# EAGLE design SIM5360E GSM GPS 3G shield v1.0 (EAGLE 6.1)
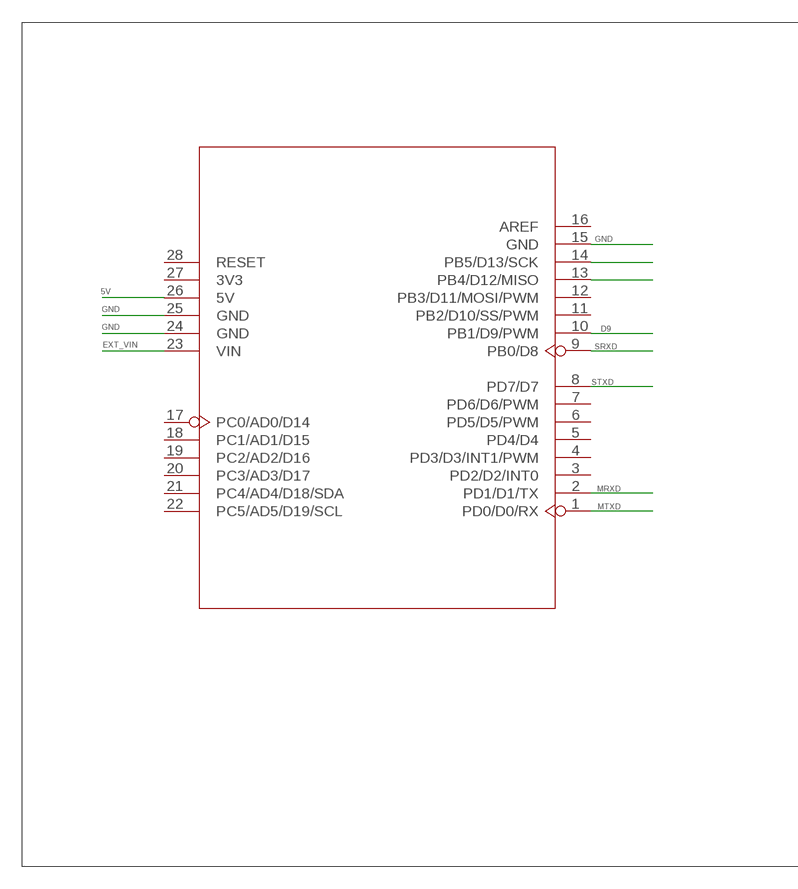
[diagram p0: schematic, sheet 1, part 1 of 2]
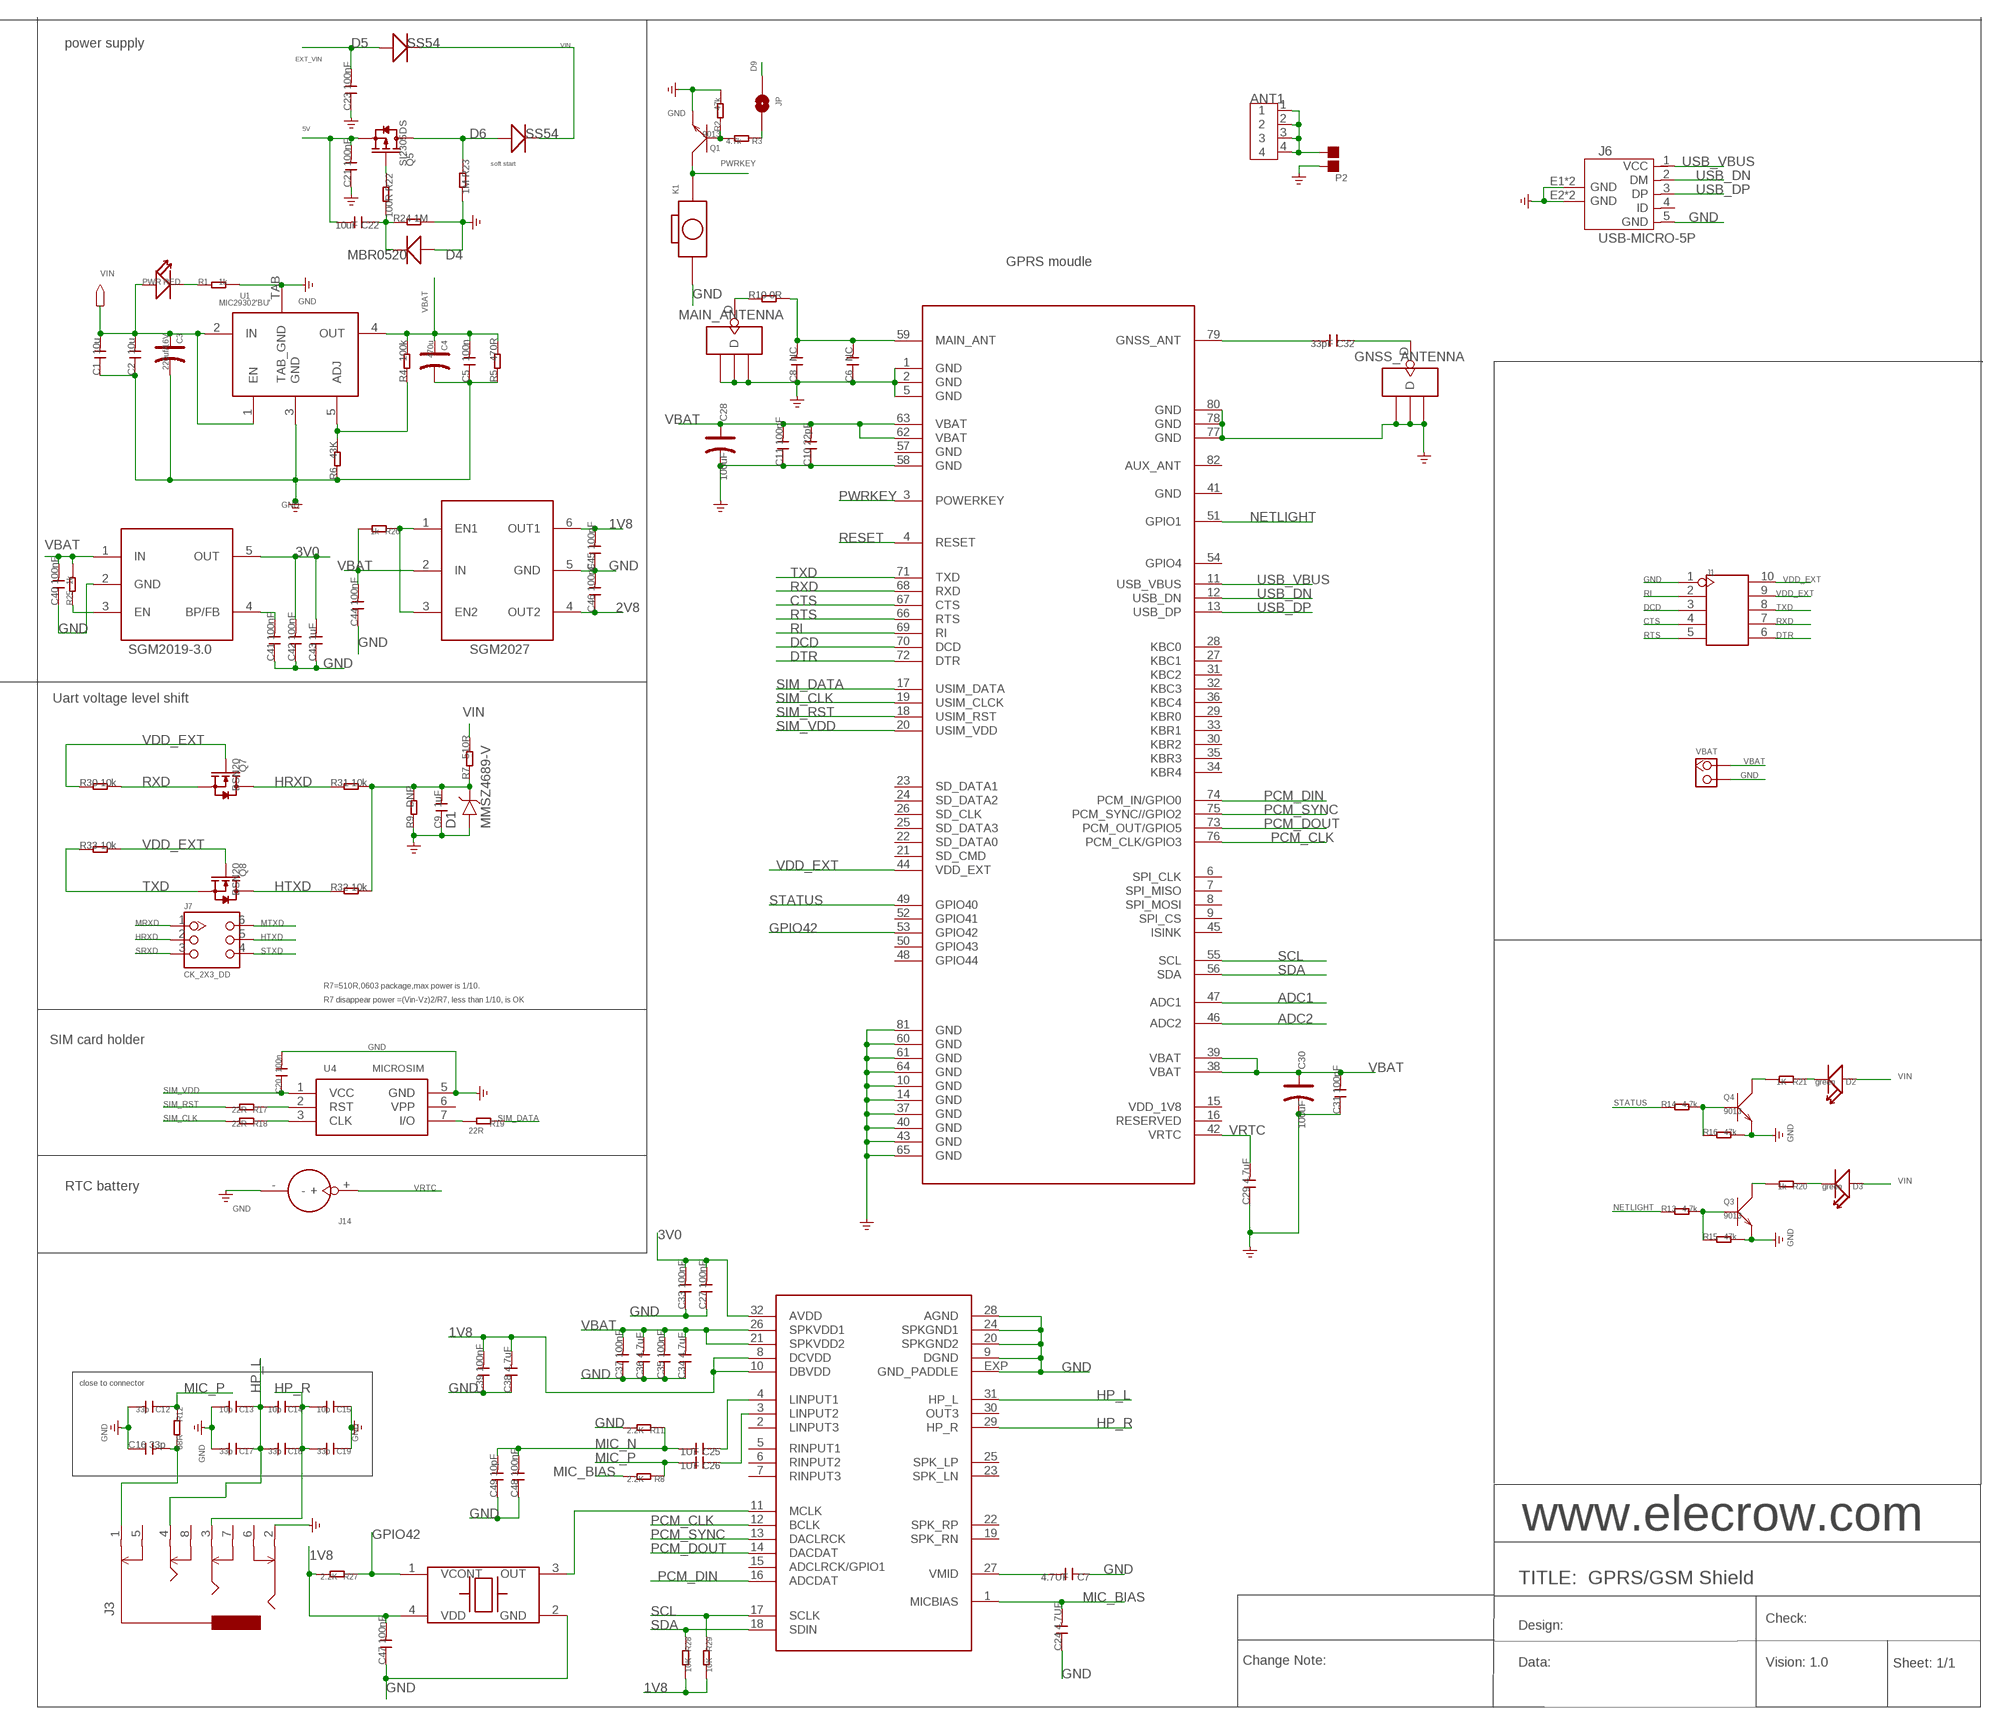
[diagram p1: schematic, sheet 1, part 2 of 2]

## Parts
ANT1  ANTENNA-SMA-IPX  [SMA-TO-IPX]
C1  10u  C-0603  [C0603]
C2  10u  C-0603  [C0603]
C3  220uf/16V  006-CAP_AVX_D  [AVX_D]
C4  470u  006-CAP_AVX_D  [AVX_D]
C5  100n  C-0603  [C0603]
C6  NC  C-0603  [C0603]
C7  4.7UF  C-0603  [C0603]
C8  NC  C-0603  [C0603]
C9  1uF  C-0603  [C0603]
C10  22pF  C-0603  [C0603]
C11  100nF  C-0603  [C0603]
C12  33p  C-0603  [C0603]
C13  10p  C-0402  [C0402]
C14  10p  C-0402  [C0402]
C15  10p  C-0402  [C0402]
C16  33p  C-0603  [C0603]
C17  33p  C-0402  [C0402]
C18  33p  C-0402  [C0402]
C19  33p  C-0402  [C0402]
C20  100n  C-0603  [C0603]
C21  100nF  C-0603  [C0603]
C22  10uF  C-0805  [C0805]
C23  100nF  C-0603  [C0603]
C24  4.7UF  C-0603  [C0603]
C25  1UF  C-0603  [C0603]
C26  1UF  C-0603  [C0603]
C27  100nF  C-0603  [C0603]
C28  100uF  CAP-AVX-B  [AVX-B]
C29  4.7uF  C-0805  [C0805]
C30  100uF  CAP-AVX-B  [AVX-B]
C31  100nF  C-0603  [C0603]
C32  33pF  C-0603  [C0603]
C33  100nF  C-0603  [C0603]
C34  4.7uF  C-0603  [C0603]
C35  100nF  C-0603  [C0603]
C36  4.7uF  C-0603  [C0603]
C37  100nF  C-0603  [C0603]
C38  4.7uF  C-0603  [C0603]
C39  100nF  C-0603  [C0603]
C40  100nF  C-0603  [C0603]
C41  100nF  C-0603  [C0603]
C42  100nF  C-0603  [C0603]
C43  1uF  C-0603  [C0603]
C44  100nF  C-0603  [C0603]
C45  100nF  C-0603  [C0603]
C46  100nF  C-0603  [C0603]
C47  100nF  C-0603  [C0603]
C48  100nF  C-0603  [C0603]
C49  10pF  C-0603  [C0603]
D1  MMSZ4689-V  D-VOL'MMSZ4681'  [SOD123-2.7X1.6]
D2  green  LED'0603'  [LED-0603]
D3  green  LED'0603'  [LED-0603]
D4  MBR0520  D'MBR0520LT1'  [SOD123-2.7X1.6]
D5  SS54  D'MBRS240LT3'  [SMB]
D6  SS54  D'MBRS240LT3'  [SMB]
GNSS_ANTENNA  ANTENNA-U-FL  [4P-U-FL]
J1  HEADER-2X5P-2.54  [2X5P-2.54]
J3  AUDIO-8P'PJ-3536-L6S'  [8P-3.5-SMD]
J6  USB-MICRO-5P  [MICRO-USB-5P]
J7  CK_2X3_DD  [CK_2X3]
J14  HOLDER-BATTERY-2P-CR1220  [CR1220]
JP  0R/0805  PAD-SOLDERJUMPERNC  [2P-SMD-3.3X2]
K1  BOTTON_1_DP  [BTN_5.0_RST]
MAIN_ANTENNA  ANTENNA-U-FL  [4P-U-FL]
P2  PAD-JUMPER-2P  [2P-SMD-1.78X1.27]
PWR  RED  007-LED0603  [D0603]
Q1  9013  TRANSISTOR-NPN-SOT23  [SOT23]
Q3  9013  TRANSISTOR-NPN-SOT23  [SOT23]
Q4  9013  TRANSISTOR-NPN-SOT23  [SOT23]
Q5  SI2305DS  MOSFET-P'SI2323CDS/SI2305DS<BR>'  [SOT23]
Q7  BSN20  MOSFET-N'SOT23'  [SOT23]
Q8  BSN20  MOSFET-N'SOT23'  [SOT23]
R1  1k  R-0603  [R0603]
R2  47k  R-0603  [R0603]
R3  4.7k  R-0603  [R0603]
R4  100k  R-0603  [R0603]
R5  470R  R-0603  [R0603]
R6  43K  R-0603  [R0603]
R7  510R  R-0603  [R0603]
R8  2.2K  R-0603  [R0603]
R9  DNP  R-0603  [R0603]
R10  0R  R-0603  [R0603]
R11  2.2K  R-0603  [R0603]
R12  68R  R-0603  [R0603]
R13  4.7k  R-0603  [R0603]
R14  4.7k  R-0603  [R0603]
R15  47k  R-0603  [R0603]
R16  47k  R-0603  [R0603]
R17  22R  R-0603  [R0603]
R18  22R  R-0603  [R0603]
R19  22R  R-0603  [R0603]
R20  1k  R-0603  [R0603]
R21  1K  R-0603  [R0603]
R22  100R  R-0603  [R0603]
R23  1M  R-0603  [R0603]
R24  1M  R-0603  [R0603]
R25  1k  R-0603  [R0603]
R26  1k  R-0603  [R0603]
R27  2.2K  R-0603  [R0603]
R28  10K  R-0603  [R0603]
R29  10K  R-0603  [R0603]
R30  10k  R-0603  [R0603]
R31  10k  R-0603  [R0603]
R32  10k  R-0603  [R0603]
R33  10k  R-0603  [R0603]
U1  MIC29302'BU'  [TO-263]
U3  UNO-SHILED  [SHILED]
U4  MICROSIM  [MICROSIM]
U5  VM8960GEFL  [QFN32-4.9X4.9]
U12  SGM2027  [TSOT6]
U21  SGM2019  [SOT23-5]
U26  8W26000011  [8W2600001]
U$8  SIM5360E  [SIM5360]
VBAT  DNP  HEADER_1X2_2.54  [CK_1*2]

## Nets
1V8: C38.2 C39.2 C45.2 C47.2 R27.2 R28.2 R29.2 U5.8(DCVDD) U5.10(DBVDD) U12.6(OUT1) U26.4(VDD)
2V8: C46.1 U12.4(OUT2)
3V0: C27.2 C33.2 C42.2 C43.2 U5.32(AVDD) U21.5(OUT)
5V: C21.2 C22.2 Q5.2(S) U3.26(5V)
ADC1: U$8.47(ADC1)
ADC2: U$8.46(ADC2)
CTS: J1.4 U$8.67(CTS)
D9: JP.1 U3.10(PB1/D9/PWM)
DCD: J1.3 U$8.70(DCD)
DTR: J1.6 U$8.72(DTR)
EXT_VIN: C23.2 D5.+ U3.23(VIN)
GND: C1.1 C2.1 C3.- C4.- C5.1 C6.1 C7.1 C8.1 C9.1 C10.1 C11.1 C12.2 C13.2 C15.1 C16.1 C17.2 C19.1 C20.2 C21.1 C23.1 C24.1 C27.1 C28.- C29.1 C30.- C31.1 C33.1 C34.1 C35.1 C36.1 C37.1 C38.1 C39.1 C40.1 C41.1 C42.1 C43.1 C44.1 C46.2 C47.1 C48.1 C49.1 D1.1 D4.1(+) GNSS_ANTENNA.GND1 GNSS_ANTENNA.GND2 GNSS_ANTENNA.GND3 J1.1 J3.2 J6.5(GND) J6.E1(GND) J6.E2(GND) J6.P1(GND) J6.P2(GND) J14.- K1.P$1 MAIN_ANTENNA.GND1 MAIN_ANTENNA.GND2 MAIN_ANTENNA.GND3 P2.2 Q1.2(E) Q3.2(E) Q4.2(E) R1.2 R2.2 R5.1 R6.1 R9.1 R11.2 R15.2 R16.2 R23.2 R24.2 U1.3(GND) U1.TAB(TAB_GND) U3.15(GND) U3.24(GND) U3.25(GND) U4.5(GND) U5.9(DGND) U5.20(SPKGND2) U5.24(SPKGND1) U5.28(AGND) U5.EXP(GND_PADDLE) U12.5(GND) U21.2(GND) U26.2(GND) U$8.1(GND) U$8.2(GND) U$8.5(GND) U$8.10(GND) U$8.14(GND) U$8.37(GND) U$8.40(GND) U$8.43(GND) U$8.58(GND) U$8.60(GND) U$8.61(GND) U$8.64(GND) U$8.65(GND) U$8.77(GND) U$8.78(GND) U$8.80(GND) U$8.81(GND) VBAT.2
GPIO42: R27.1 U26.1(VCONT) U$8.53(GPIO42)
HP_L: C13.1 C14.2 C17.1 C18.2 J3.4 U5.31(HP_L)
HP_R: C14.1 C15.2 C18.1 C19.2 J3.3 U5.29(HP_R)
HRXD: J7.2 Q7.3(D) R31.1
HTXD: J7.5 Q8.3(D) R32.1
MIC_BIAS: C24.2 R8.2 U5.1(MICBIAS)
MIC_N: C25.2 C48.2 C49.2 R11.1
MIC_P: C12.1 C26.2 R8.1 R12.1
MRXD: J7.1 U3.2(PD1/D1/TX)
MTXD: J7.6 U3.1(PD0/D0/RX)
N$1: R19.2 U4.7(I/O)
N$2: R4.1 R6.2 U1.5(ADJ)
N$3: Q3.3(C) R20.2
N$4: C7.2 U5.27(VMID)
N$5: R18.1 U4.3(CLK)
N$6: R17.1 U4.2(RST)
N$7: D3.- R20.1
N$8: Q3.1(B) R13.2 R15.1
N$9: C9.2 D1.2 R7.1 R9.2 R31.2 R32.2
N$11: Q5.1(G) R22.1
N$12: ANT1.1 ANT1.2 ANT1.3 ANT1.4 P2.1
N$13: U5.11(MCLK) U26.3(OUT)
N$14: JP.2 R3.1
N$15: C6.2 C8.2 R10.2 U$8.59(MAIN_ANT)
N$16: Q4.3(C) R21.2
N$17: D2.- R21.1
N$18: Q4.1(B) R14.2 R16.1
N$19: MAIN_ANTENNA.D R10.1
N$20: D6.+ Q5.3(D) R23.1
N$21: C25.1 U5.4(LINPUT1)
N$22: C26.1 U5.3(LINPUT2)
N$23: U3.14(PB5/D13/SCK)
N$25: C41.2 U21.4(BP/FB)
N$26: R25.1 U21.3(EN)
N$27: U3.13(PB4/D12/MISO)
N$28: R26.1 U12.1(EN1) U12.3(EN2)
N$30: C16.2 J3.1 R12.2
N$36: Q1.1(B) R2.1 R3.2
N$39: C22.1 D4.2(-) R22.2 R24.1
N$53: PWR.- R1.1
N$54: C32.2 U$8.79(GNSS_ANT)
N$55: C32.1 GNSS_ANTENNA.D
NETLIGHT: R13.1 U$8.51(GPIO1)
PCM_CLK: U5.12(BCLK) U$8.76(PCM_CLK/GPIO3)
PCM_DIN: U5.16(ADCDAT) U$8.74(PCM_IN/GPIO0)
PCM_DOUT: U5.14(DACDAT) U$8.73(PCM_OUT/GPIO5)
PCM_SYNC: U5.13(DACLRCK) U$8.75(PCM_SYNC//GPIO2)
PWRKEY: K1.P$2 Q1.3(C) U$8.3(POWERKEY)
RESET: U$8.4(RESET)
RI: J1.2 U$8.69(RI)
RTS: J1.5 U$8.66(RTS)
RXD: J1.7 Q7.2(S) R30.2 U$8.68(RXD)
SCL: R29.1 U5.17(SCLK) U$8.55(SCL)
SDA: R28.1 U5.18(SDIN) U$8.56(SDA)
SIM_CLK: R18.2 U$8.19(USIM_CLCK)
SIM_DATA: R19.1 U$8.17(USIM_DATA)
SIM_RST: R17.2 U$8.18(USIM_RST)
SIM_VDD: C20.1 U4.1(VCC) U$8.20(USIM_VDD)
SRXD: J7.3 U3.9(PB0/D8)
STATUS: R14.1 U$8.49(GPIO40)
STXD: J7.4 U3.8(PD7/D7)
TXD: J1.8 Q8.2(S) R33.1 U$8.71(TXD)
USB_DN: J6.2(DM) U$8.12(USB_DN)
USB_DP: J6.3(DP) U$8.13(USB_DP)
USB_VBUS: J6.1(VCC) U$8.11(USB_VBUS)
VBAT: C4.+ C5.2 C10.2 C11.2 C28.+ C30.+ C31.2 C34.2 C35.2 C36.2 C37.2 C40.2 C44.2 R4.2 R5.2 R25.2 R26.2 U1.4(OUT) U5.21(SPKVDD2) U5.26(SPKVDD1) U12.2(IN) U21.1(IN) U$8.38(VBAT) U$8.39(VBAT) U$8.62(VBAT) U$8.63(VBAT) VBAT.1
VDD_EXT: J1.9 J1.10 Q7.1(G) Q8.1(G) R30.1 R33.2 U$8.44(VDD_EXT)
VIN: C1.2 C2.2 C3.+ D2.+ D3.+ D5.- D6.- PWR.+ R7.2 U1.1(EN) U1.2(IN)
VRTC: C29.2 J14.+ U$8.42(VRTC)
Unconnected: C45.1 J3.5 J3.6 J3.7 J3.8 J6.4(ID) U3.3(PD2/D2/INT0) U3.4(PD3/D3/INT1/PWM) U3.5(PD4/D4) U3.6(PD5/D5/PWM) U3.7(PD6/D6/PWM) U3.11(PB2/D10/SS/PWM) U3.12(PB3/D11/MOSI/PWM) U3.16(AREF) U3.17(PC0/AD0/D14) U3.18(PC1/AD1/D15) U3.19(PC2/AD2/D16) U3.20(PC3/AD3/D17) U3.21(PC4/AD4/D18/SDA) U3.22(PC5/AD5/D19/SCL) U3.27(3V3) U3.28(RESET) U4.6(VPP) U5.2(LINPUT3) U5.5(RINPUT1) U5.6(RINPUT2) U5.7(RINPUT3) U5.15(ADCLRCK/GPIO1) U5.19(SPK_RN) U5.22(SPK_RP) U5.23(SPK_LN) U5.25(SPK_LP) U5.30(OUT3) U$8.6(SPI_CLK) U$8.7(SPI_MISO) U$8.8(SPI_MOSI) U$8.9(SPI_CS) U$8.15(VDD_1V8) U$8.16(RESERVED) U$8.21(SD_CMD) U$8.22(SD_DATA0) U$8.23(SD_DATA1) U$8.24(SD_DATA2) U$8.25(SD_DATA3) U$8.26(SD_CLK) U$8.27(KBC1) U$8.28(KBC0) U$8.29(KBR0) U$8.30(KBR2) U$8.31(KBC2) U$8.32(KBC3) U$8.33(KBR1) U$8.34(KBR4) U$8.35(KBR3) U$8.36(KBC4) U$8.41(GND) U$8.45(ISINK) U$8.48(GPIO44) U$8.50(GPIO43) U$8.52(GPIO41) U$8.54(GPIO4) U$8.57(GND) U$8.82(AUX_ANT)

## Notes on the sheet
- power supply
- soft start
- GPRS moudle
- SGM2019-3.0 | SGM2027
- Uart voltage level shift
- R7=510R,0603 package,max power is 1/10.
- R7 disappear power =(Vin-Vz)2/R7, less than 1/10, is OK
- SIM card holder
- RTC battery
- close to connector
- www.elecrow.com
- TITLE:  GPRS/GSM Shield
- Check:
- Design:
- Change Note: | Data: | Vision: 1.0 | Sheet: 1/1

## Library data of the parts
ANT1 = Connector:ANTENNA-SMA-IPX
C1 C2 C5-C27 C29 C31-C49 = Discrete:C*: Ceramic Capacitors
C3 C4 = Discrete:006-CAP*: Electrolytic Capacitors,Tantalum Capacitors and Super Capacitors
C28 C30 = Discrete:CAP*: Electrolytic Capacitors,Tantalum Capacitors and Super Capacitors
D1 = template:D-VOL
D2 D3 = Discrete:LED*
D4-D6 = Discrete:D*
GNSS_ANTENNA MAIN_ANTENNA = Connector:ANTENNA-U-FL
J1 = Connector:HEADER-2X5P
J3 = template:AUDIO-8P
J6 = Connector:USB-MICRO-5P
J7 = CONNECTER:CK_2X3
J14 = Connector:HOLDER-BATTERY-2P
JP = Discrete:PAD-SOLDERJUMPER: Solder Jumper
K1 = CPT_SMD:BOTTON_1
P2 = Discrete:PAD-JUMPER-2P; PARTNO: DNP
PWR = Discrete:007-LED*
Q1 Q3 Q4 = Discrete:TRANSISTOR-NPN*: NPN audion
Q5 = Discrete:MOSFET-P
Q7 Q8 = Discrete:MOSFET-N: IRLL014: http://www.vishay.com/docs/91319/sihll014.pdf
R1-R33 = Discrete:R*
U1 = ICs_v54:MIC29302
U3 = ljb:UNO-SHILED
U4 = Connector:MICROSIM
U5 = IC:VM8960GEFL
U12 = IC:SGM2027
U21 = IC:SGM2019
U26 = Discrete:8W26000011
U$8 = IC:SIM5360E
VBAT = CONNECTER:HEADER_1X2

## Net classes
0 default: width 0.152 mm, drill 0.152 mm, clearance 0.152 mm

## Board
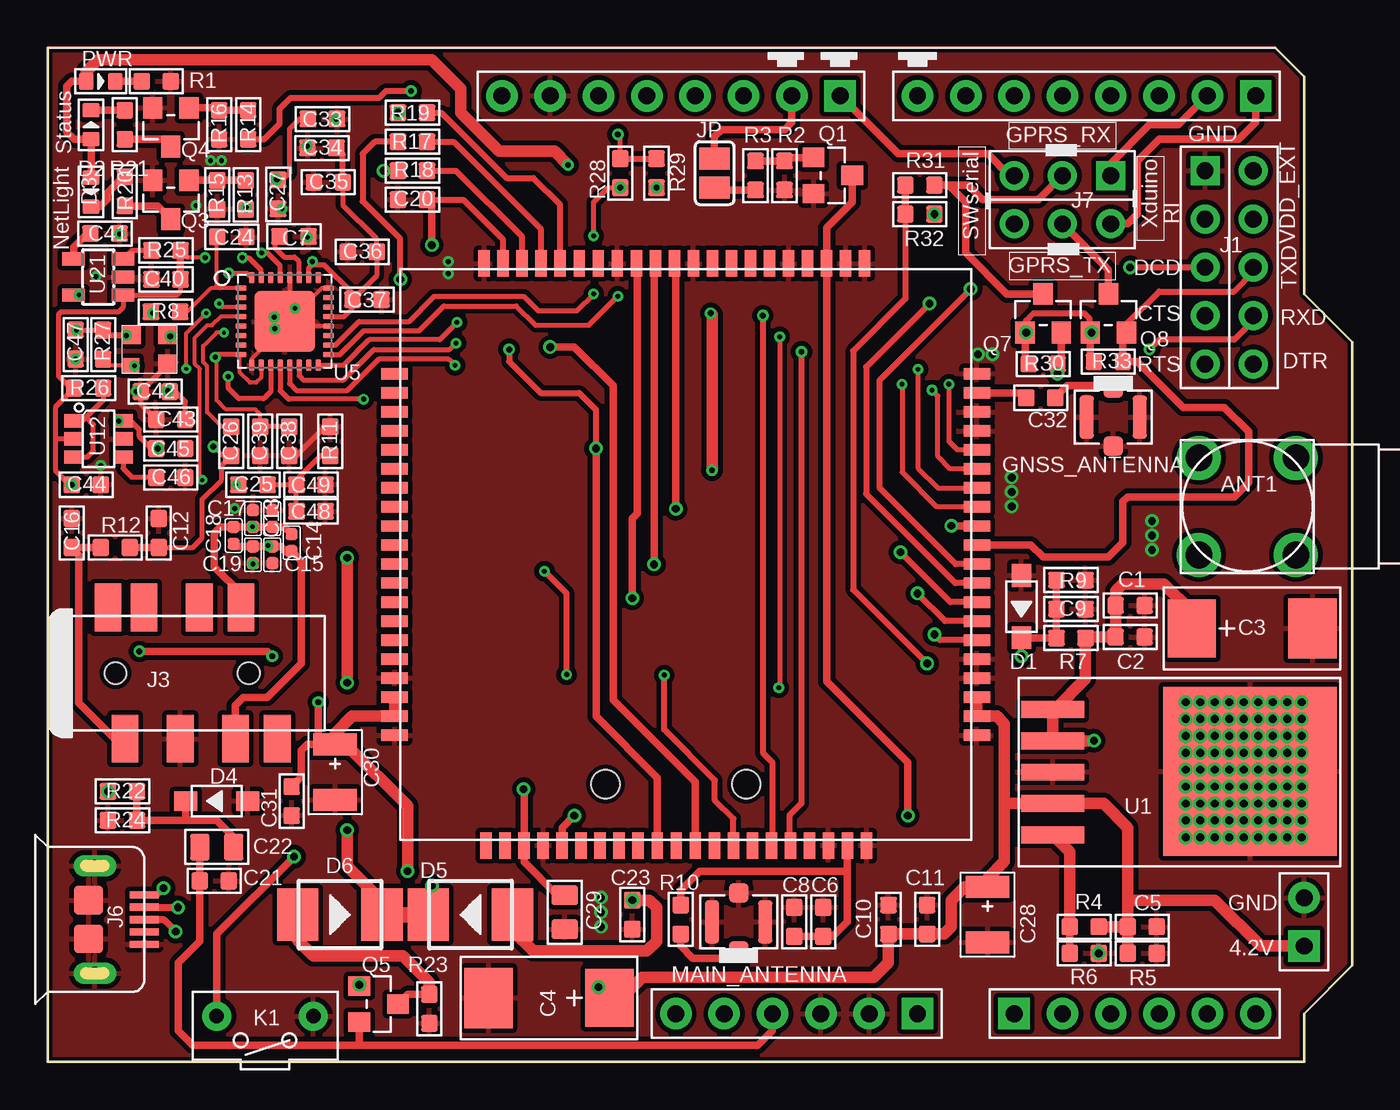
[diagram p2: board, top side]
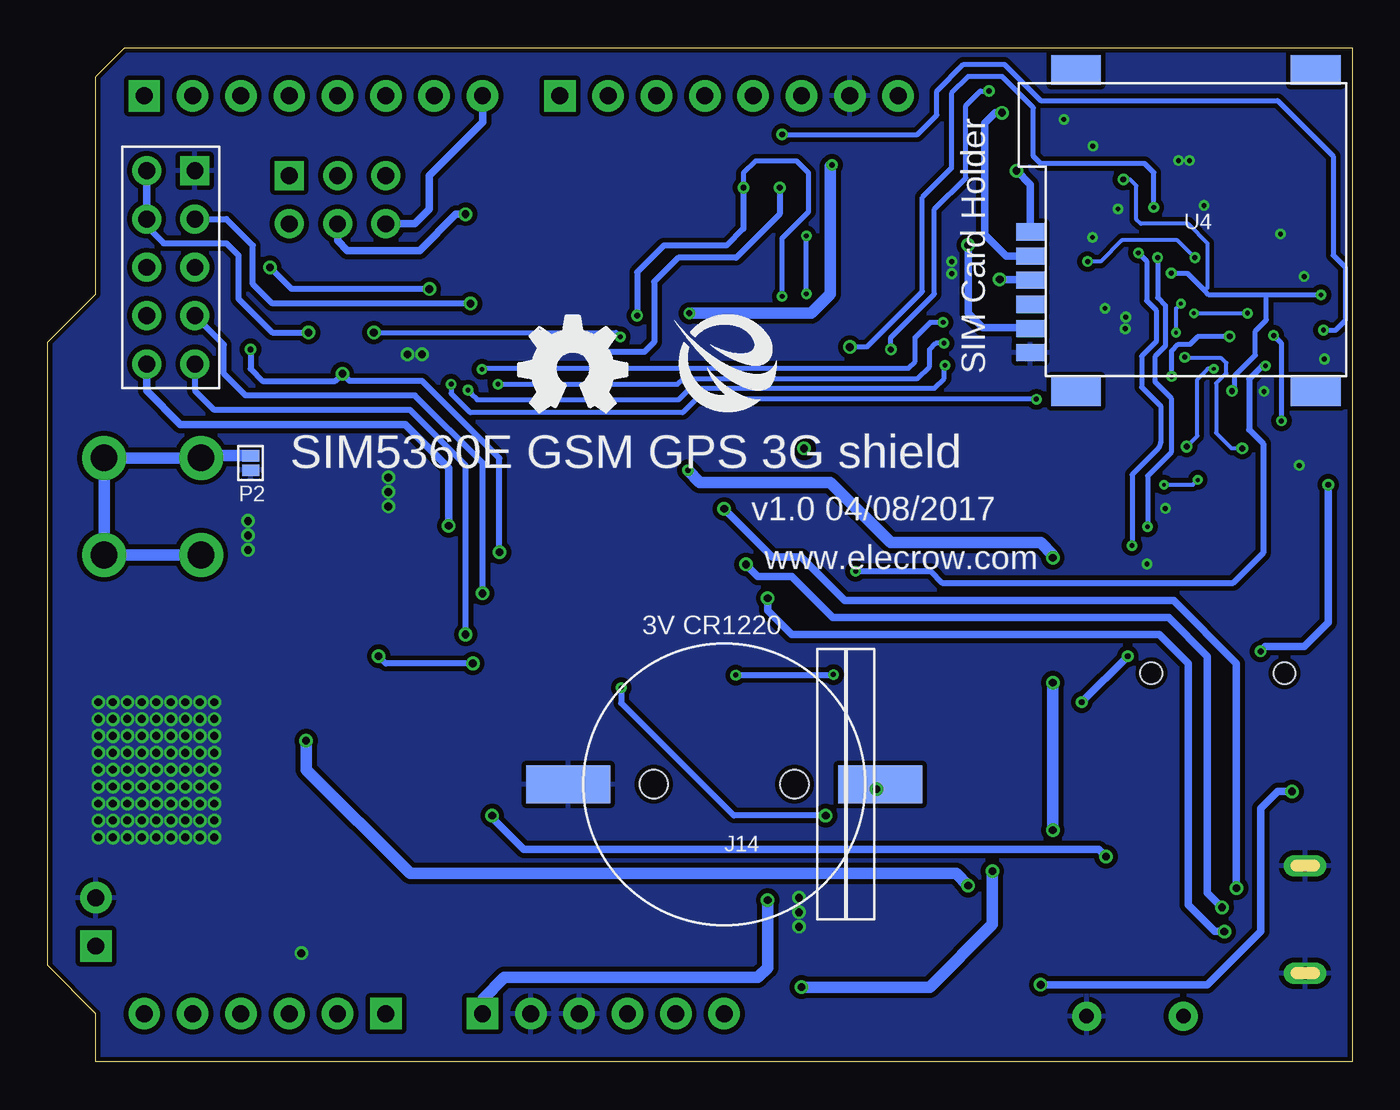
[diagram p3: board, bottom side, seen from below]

Size 68.58 x 53.34 mm. Coordinates in mm from the lower left corner, seen from the top.
Outline: 64.52,53.34 0,53.34 0,0 66.04,0 66.04,2.54 68.58,5.08 68.58,37.85 66.04,40.39 66.04,51.82 64.52,53.34
Copper layers (1*16): Top 0.035mm / dielectric 1.5mm / Bottom 0.035mm
Design rules: minimum track width 6mil, minimum drill 7mil, track to track 6mil, track to pad 6mil, pad to pad 6mil, via to via 6mil, smd to smd 0mil, copper to edge 10mil, drill to drill 10mil, minimum pad ring 10mil, minimum via ring 6mil, stop-mask expansion 2mil, vias tented up to drill 100mil, thermal gap 10mil
tRestrict: 1 lines

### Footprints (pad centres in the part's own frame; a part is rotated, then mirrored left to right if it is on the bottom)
SMA-TO-IPX = drill 1.4 pad 2.3: 1 -2.55,2.55; 2 2.55,2.55; 3 2.55,-2.55; 4 -2.55,-2.55
C0603 = smd 0.889 x 0.889: 1 -0.762,0; 2 0.762,0
AVX_D = smd 2.54 x 3.048: + -3.175,0 | smd 2.54 x 3.175: - 3.175,0
C0402 = smd 0.635 x 0.635: 1 -0.445,0; 2 0.445,0
C0805 = smd 1.016 x 1.397: 1 -0.889,0; 2 0.889,0
AVX-B = smd 1.143 x 2.286: + -1.46,0; - 1.46,0
SOD123-2.7X1.6 = smd 1.2 x 1.02: 1 -1.635,0; 2 1.635,0
D0603 = smd 0.762 x 0.889: + -0.762,0; - 0.762,0
SMB = smd 2.159 x 2.743: + -2.21,0; - 2.21,0
4P-U-FL = smd 1.016 x 1.016: D -1.524,0; GND3 1.524,0 | smd 2.286 x 0.762: GND1 0,1.397; GND2 0,-1.397
2X5P-2.54-LEADED = drill 0.889 pad 1.524 square: 1 -1.27,5.08 | drill 0.889 pad 1.524: 2 -1.27,2.54; 3 -1.27,0; 4 -1.27,-2.54; 5 -1.27,-5.08; 6 1.27,-5.08; 7 1.27,-2.54; 8 1.27,0; 9 1.27,2.54; 10 1.27,5.08
8P-3.5-SMD = smd 1.4 x 2.5: 1 2.8,-3.45; 2 5.7,-3.45; 3 8.6,-3.45; 4 8.9,3.45; 5 1.9,3.45; 6 3.8,3.45; 7 6.7,3.45; 8 10.8,-3.45 | hole 1.149: 2.3,0; 9.3,0
MICRO-USB-5P = smd 0.38 x 1.52: 1 -1.3,0; 2 -0.65,0; 3 0,0; 4 0.65,0; 5 1.3,0 | smd 1.524 x 1.524: E1 -1.016,-2.921; E2 1.016,-2.921 | drill 0.635 pad 1.143 long: P1 -2.819,-2.591; P2 2.819,-2.591
CK_2X3 = drill 0.889 pad 1.524 square: 1 -1.27,2.54 | drill 0.889 pad 1.524: 2 -1.27,0; 3 -1.27,-2.54; 4 1.27,-2.54; 5 1.27,0; 6 1.27,2.54
CR1220 = smd 2 x 4.4: + 0,-8.2; - 0,8.2 | hole 1.5: 0,3.7; 0,-3.7
2P-SMD-3.3X2 = smd 1.168 x 1.6: 1 -0.762,0; 2 0.762,0
BTN_5.0_RST = drill 0.762 pad 1.524: P$1 0,2.54; P$2 0,-2.54
2P-SMD-1.78X1.27 = smd 0.889 x 0.61: 1 0,0.381; 2 0,-0.381
SOT23 = smd 1.016 x 1.143: 1 -0.95,-1.016; 2 0.95,-1.016; 3 0,1.016
R0603 = smd 0.889 x 0.889: 1 -0.762,0; 2 0.762,0
TO-263 = smd 3.302 x 0.889: 1 3.302,-3.302; 2 3.302,-1.651; 3 3.302,0; 4 3.302,1.651; 5 3.302,3.302 | smd 9.12 x 8.89: TAB -7.071,-0.03
SHILED = drill 0.889 pad 1.651 square: 1 63.5,50.8; 9 41.656,50.8; 17 50.8,2.54; 23 45.72,2.54 | drill 0.889 pad 1.651: 2 60.96,50.8; 3 58.42,50.8; 4 55.88,50.8; 5 53.34,50.8; 6 50.8,50.8; 7 48.26,50.8; 8 45.72,50.8; 10 39.116,50.8; 11 36.576,50.8; 12 34.036,50.8; 13 31.496,50.8; 14 28.956,50.8; 15 26.416,50.8; 16 23.876,50.8; 18 53.34,2.54; 19 55.88,2.54; 20 58.42,2.54; 21 60.96,2.54; 22 63.5,2.54; 24 43.18,2.54; 25 40.64,2.54; 26 38.1,2.54; 27 35.56,2.54; 28 33.02,2.54
MICROSIM = smd 1.5 x 0.9: 1 -0.8,2.5; 2 -0.8,5.04; 3 -0.8,7.58; 5 -0.8,1.23; 6 -0.8,3.77; 7 -0.8,6.31 | smd 2.61 x 1.56: P$1 1.6,-0.8; P$2 14.2,-0.8; P$3 14.2,16.1; P$4 1.6,16.1
QFN32-4.9X4.9 = smd 0.6 x 0.3: 1 -2.3,1.75; 2 -2.3,1.25; 3 -2.3,0.75; 4 -2.3,0.25; 5 -2.3,-0.25; 6 -2.3,-0.75; 7 -2.3,-1.25; 8 -2.3,-1.75; 17 2.3,-1.75; 18 2.3,-1.25; 19 2.3,-0.75; 20 2.3,-0.25; 21 2.3,0.25; 22 2.3,0.75; 23 2.3,1.25; 24 2.3,1.75 | smd 0.3 x 0.6: 9 -1.75,-2.3; 10 -1.25,-2.3; 11 -0.75,-2.3; 12 -0.25,-2.3; 13 0.25,-2.3; 14 0.75,-2.3; 15 1.25,-2.3; 16 1.75,-2.3; 25 1.75,2.3; 26 1.25,2.3; 27 0.75,2.3; 28 0.25,2.3; 29 -0.25,2.3; 30 -0.75,2.3; 31 -1.25,2.3; 32 -1.75,2.3 | smd 3.2 x 3.2: EXP 0,0
TSOT6 = smd 0.69 x 1: 1 -0.95,-1.3; 2 0,-1.3; 3 0.95,-1.3; 4 0.95,1.3; 5 0,1.3; 6 -0.95,1.3
SOT23-5 = smd 0.69 x 1.2: 1 -0.95,-1.3; 2 0,-1.3; 3 0.95,-1.3; 4 0.95,1.3; 5 -0.95,1.3
8W2600001 = smd 0.9 x 0.8: 1 -1,-0.85 | smd 1 x 0.95: 2 0.95,-0.75; 3 0.95,0.75; 4 -0.95,0.75
SIM5360 = smd 0.6 x 1.4: 1 24.4,30.3; 2 23.4,30.3; 3 22.4,30.3; 4 21.4,30.3; 5 20.4,30.3; 6 19.4,30.3; 7 18.4,30.3; 8 17.4,30.3; 9 16.4,30.3; 10 15.4,30.3; 11 14.4,30.3; 12 13.4,30.3; 13 12.4,30.3; 14 11.4,30.3; 15 10.4,30.3; 16 9.4,30.3; 17 8.4,30.3; 18 7.4,30.3; 19 6.4,30.3; 20 5.4,30.3; 41 5.5,-0.3; 42 6.5,-0.3; 43 7.5,-0.3; 44 8.5,-0.3; 45 9.5,-0.3; 46 10.5,-0.3; 47 11.5,-0.3; 48 12.5,-0.3; 49 13.5,-0.3; 50 14.5,-0.3; 51 15.5,-0.3; 52 16.5,-0.3; 53 17.5,-0.3; 54 18.5,-0.3; 55 19.5,-0.3; 56 20.5,-0.3; 57 21.5,-0.3; 58 22.5,-0.3; 59 23.5,-0.3; 60 24.5,-0.3; 81 4.4,30.3; 82 4.5,-0.3 | smd 1.4 x 0.6: 21 -0.3,24.5; 22 -0.3,23.5; 23 -0.3,22.5; 24 -0.3,21.5; 25 -0.3,20.5; 26 -0.3,19.5; 27 -0.3,18.5; 28 -0.3,17.5; 29 -0.3,16.5; 30 -0.3,15.5; 31 -0.3,14.5; 32 -0.3,13.5; 33 -0.3,12.5; 34 -0.3,11.5; 35 -0.3,10.5; 36 -0.3,9.5; 37 -0.3,8.5; 38 -0.3,7.5; 39 -0.3,6.5; 40 -0.3,5.5; 61 30.3,5.5; 62 30.3,6.5; 63 30.3,7.5; 64 30.3,8.5; 65 30.3,9.5; 66 30.3,10.5; 67 30.3,11.5; 68 30.3,12.5; 69 30.3,13.5; 70 30.3,14.5; 71 30.3,15.5; 72 30.3,16.5; 73 30.3,17.5; 74 30.3,18.5; 75 30.3,19.5; 76 30.3,20.5; 77 30.3,21.5; 78 30.3,22.5; 79 30.3,23.5; 80 30.3,24.5
CK_1*2 = drill 0.889 pad 1.651 square: 1 0,1.27 | drill 0.889 pad 1.651: 2 0,-1.27

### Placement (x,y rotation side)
ANT1  63.06,29.21 90 top
C1  56.9,24 180 top
C2  56.9,22.35 180 top
C3  63.31,22.8 0 top
C4  26.35,3.37 180 top
C5  57.53,7.11 180 top
C6  40.77,7.37 270 top
C7  12.95,43.41 180 top
C8  39.24,7.37 270 top
C9  53.78,23.81 180 top
C10  44.2,7.49 270 top
C11  46.23,7.49 270 top
C12  5.84,27.81 90 top
C13  11.81,28.57 90 top
C14  12.83,27.3 90 top
C15  11.81,26.67 90 top
C16  1.27,27.81 270 top
C17  10.79,28.57 90 top
C18  9.78,27.69 90 top
C19  10.79,26.67 90 top
C20  19.18,45.34 180 top
C21  8.76,9.53 180 top
C22  8.89,11.3 180 top
C23  30.73,7.75 90 top
C24  9.68,43.38 180 top
C25  10.79,30.35 0 top
C26  9.65,32.64 270 top
C27  12.12,45.62 90 top
C28  49.4,7.75 270 top
C29  27.18,7.87 90 top
C30  15.11,15.24 270 top
C31  12.83,13.72 90 top
C32  52.2,34.92 180 top
C33  14.45,49.58 180 top
C34  14.43,48.06 0 top
C35  14.76,46.25 0 top
C36  16.54,42.6 0 top
C37  16.79,40.08 180 top
C38  12.7,32.64 90 top
C39  11.18,32.64 90 top
C40  6.22,41.15 0 top
C41  3.02,43.56 180 top
C42  5.66,35.26 0 top
C43  6.48,33.78 0 top
C44  2.03,30.35 180 top
C45  6.48,32.26 180 top
C46  6.48,30.73 0 top
C47  1.47,37.72 90 top
C48  13.84,28.96 180 top
C49  13.84,30.35 180 top
D1  51.18,23.94 270 top
D2  green  [D0603]  2.29,49.28 90 top
D3  green  [D0603]  2.29,45.75 270 top
D4  8.89,13.72 180 top
D5  22.23,7.75 180 top
D6  15.37,7.75 0 top
GNSS_ANTENNA  56.01,33.91 270 top
J1  [2X5P-2.54-LEADED]  62.1,41.78 0 top
J3  1.27,20.45 0 top
J6  5.08,7.49 270 top
J7  53.34,45.34 270 top
J14  33.02,14.61 90 bottom
JP  35.05,46.74 270 top
K1  11.43,2.41 270 top
LOGO2  LOGO-OSHW-FILLX0200-NT  [OSHW_FILLX200_NOTEXT]  43.81,34.16 0 bottom
MAIN_ANTENNA  36.32,7.37 90 top
P2  57.91,31.5 0 bottom
PWR  2.79,51.56 0 top
Q1  41.27,46.61 270 top
Q3  6.48,45.34 180 top
Q4  6.48,49.15 180 top
Q5  17.4,3.05 270 top
Q7  52.32,39.37 0 top
Q8  55.75,39.37 0 top
R1  5.71,51.56 0 top
R2  38.73,46.61 270 top
R3  37.21,46.61 90 top
R4  54.48,7.11 0 top
R5  57.53,5.71 180 top
R6  54.48,5.71 180 top
R7  53.78,22.29 0 top
R8  6.2,39.45 0 top
R9  53.78,25.34 180 top
R10  33.27,7.49 90 top
R11  14.86,32.64 90 top
R12  3.56,27.05 180 top
R13  10.41,45.59 90 top
R14  10.54,49.28 90 top
R15  8.92,45.59 270 top
R16  9.02,49.28 270 top
R17  19.18,48.39 0 top
R18  19.18,46.86 0 top
R19  19.18,49.91 180 top
R20  4.06,45.77 270 top
R21  4.06,49.28 270 top
R22  3.94,14.22 0 top
R23  20.07,2.79 270 top
R24  3.94,12.7 180 top
R25  6.22,42.67 0 top
R26  2.16,35.43 180 top
R27  2.92,37.72 90 top
R28  30.1,46.74 90 top
R29  32,46.74 90 top
R30  52.32,36.7 0 top
R31  45.85,46.1 180 top
R32  45.85,44.58 180 top
R33  55.75,36.83 180 top
U1  56.13,15.24 180 top
U3  0,0 0 top
U4  16.13,36.07 0 bottom
U5  12.47,38.94 0 top
U12  2.67,32.77 270 top
U21  2.67,41.27 90 top
U26  5.36,37.47 0 top
U$1  [ELECROW-NEW]  35.69,34.16 0 bottom
U$8  18.54,11.68 0 top
VBAT  66.04,7.37 180 top

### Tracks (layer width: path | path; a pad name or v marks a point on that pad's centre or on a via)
1V8  (via drill 0.25, 0.3)
  Top 0.203: C39.2 11.18,34.06 10.92,34.31 9.37,34.31 8.89,34.8 8.89,36.98 | U5.10 11.22,35.99 10.95,35.71 10.64,35.71 10.11,36.25 10.11,37.13 U5.8
  Top 0.254: 3.19,38.22 R27.2 v1.52,38.48 C47.2 | C45.2 5.46,32.26 4.83,32.89 4.83,33.25 4.37,33.71 3.98,33.71 U12.6 3.74,33.72 v3.73,33.71 | C38.2 C39.2 | U5.8 8.94,37.19 v8.81,37.06 8.89,36.98 | v4.14,38.2 4.4,38.2 U26.4 | R28.2 30.1,48.64 v29.97,48.77
  Top 0.305: v4.14,38.2 3.2,38.2 R27.2 | C45.2 v5.79,32.26 | R28.2 R29.2
  Bottom 0.203: 8.76,37.01 6.88,37.01 6.63,36.75 6.63,36.22 7.16,35.69 7.16,33.07 6.35,32.26 v5.79,32.26
  Bottom 0.254: v3.73,33.71 3.73,37.8 v4.14,38.2 | 8.76,37.01 v8.81,37.06 | v29.97,48.77 22.86,48.77 21.84,49.78 21.84,51.05 20.45,52.45 18.29,52.45 16.38,50.55 3.94,50.55 1.02,47.62 1.02,42.42 0.38,41.78 0.38,38.99 0.89,38.48 v1.52,38.48
2V8
  Top 0.254: U12.4 3.97,31.21 4.45,30.73 C46.1
3V0  (via drill 0.25, 0.3)
  Top 0.203: C27.2 12.06,46.38 v12.04,46.41
  Top 0.254: 1.39,40.33 U21.5 1.38,40.34 v1.65,40.34 | C33.2 13.23,49.58 12.72,49.07 12.72,46.74 12.37,46.38 C27.2 | v9.53,41.48 10.48,41.48 U5.32 | C43.2 7.24,34.72 6.71,35.26 C42.2 6.35,35.26 v6.33,35.28
  Bottom 0.203: 7.77,40.56 7.62,40.72 7.62,43.05 8.64,44.07 11.12,44.07 11.35,44.3 11.35,46.08 11.68,46.41 v12.04,46.41
  Bottom 0.254: v1.65,40.34 4.52,40.34 | 4.52,40.34 7.54,40.34 7.77,40.56 8.69,41.48 v9.53,41.48 | 4.52,40.34 4.52,39.01 5.11,38.43 5.11,37.16 6.17,36.09 6.17,35.43 v6.33,35.28
5V
  Top 0.406: C22.2 C21.2 8,6.35 6.86,5.21 6.86,1.65 7.62,0.89 16.51,0.89 | U3.26 38.1,1.65 37.34,0.89 16.51,0.89 | Q5.2 16.38,1.02 16.51,0.89
CTS  (via drill 0.41)
  Top 0.305: U$8.67 47.17,23.18 v45.72,24.64
  Bottom 0.305: v45.72,24.64 45.72,31.5 49.28,35.05 58.17,35.05 59.31,36.2 59.31,37.72 J1.4
D9
  Top 0.406: JP.1 35.05,48.64 35.43,49.02 38.73,49.02 39.12,49.4 U3.10
DCD  (via drill 0.41)
  Top 0.305: U$8.70 47.73,26.18 43.71,30.2 43.71,35.84 v48.51,40.64 | v56.9,41.78 J1.3
  Bottom 0.305: v48.51,40.64 55.75,40.64 v56.9,41.78
DTR  (via drill 0.41)
  Top 0.406: U$8.72 v47.51,28.18 v47.5,28.19
  Bottom 0.406: v47.5,28.19 47.5,31.24 49.78,33.53 61.59,33.53 63.37,35.31 J1.6
EXT_VIN  (via drill 0.41)
  Top 0.61: D5.+ 24.43,6.93 25.53,5.84 31.5,5.84 32,6.35 32,8.13 31.62,8.51 C23.2
  Bottom 0.61: U3.23 45.72,3.3 44.58,4.45 31.24,4.45 30.73,4.95 C23.2
  other vias: 30.73,8.51
GND  (via drill 0.25, 0.41)
  Top 0.203: U5.24 14.4,40.69 13.72,40.01 13.72,38.96 13.99,38.69 U5.20 | U5.9 10.72,36.98 11.94,38.2 v11.94,38.56 | v11.91,39.17 11.91,39.22 11.94,39.24
  Top 0.254: C38.1 13.08,31.88 14.61,33.4 R11.2 | 11.94,39.24 11.93,39.25 12.17,39.25 | U5.28 12.72,39.91 v13.01,39.62 | v13.01,39.62 13.01,39.47 U5.EXP | 13.72,40.01 13.39,40.01 v13.01,39.62 | v11.94,38.56 11.94,38.18 | U26.2 6.31,36.66 C42.1 4.9,34.59 C43.1
  other vias: 55.24,5.71 58.04,28.45 58.04,27.69 58.04,26.92 50.67,29.97 50.67,29.21 50.67,30.73 29.08,8.64 29.08,7.87 29.08,7.11 59.82,18.92 60.58,18.92 61.34,18.92 62.1,18.92 62.87,18.92 63.63,18.92 64.39,18.92 65.15,18.92 65.91,18.92 59.82,18.03 60.58,18.03 61.34,18.03 62.1,18.03 62.87,18.03 63.63,18.03 64.39,18.03 65.15,18.03 65.91,18.03 59.82,17.14 60.58,17.14 61.34,17.14 62.1,17.14 62.87,17.14 63.63,17.14 64.39,17.14 65.15,17.14 65.91,17.14 59.82,16.26 60.58,16.26 61.34,16.26 62.1,16.26 62.87,16.26 63.63,16.26 64.39,16.26 65.15,16.26 65.91,16.26 59.82,15.37 60.58,15.37 61.34,15.37 62.1,15.37 62.87,15.37 63.63,15.37 64.39,15.37 65.15,15.37 65.91,15.37 59.82,14.48 60.58,14.48 61.34,14.48 62.1,14.48 62.87,14.48 63.63,14.48 64.39,14.48 65.15,14.48 65.91,14.48 59.82,13.59 60.58,13.59 61.34,13.59 62.1,13.59 62.87,13.59 63.63,13.59 64.39,13.59 65.15,13.59 65.91,13.59 59.82,12.7 60.58,12.7 61.34,12.7 62.1,12.7 62.87,12.7 63.63,12.7 64.39,12.7 65.15,12.7 65.91,12.7 59.82,11.81 60.58,11.81 61.34,11.81 62.1,11.81 62.87,11.81 63.63,11.81 64.39,11.81 65.15,11.81 65.91,11.81 2.54,41.3 1.47,36.96 3.78,43.54 7.8,45.03 13.67,43.36 9.83,29.11 10.79,26.19 48.9,37.21 49.66,37.21 2.79,31.37 4.65,35.26 12.32,44.86 8.56,47.4 9.14,47.4 13.64,48.16 15.16,49.56 21.06,42.09 21.06,41.45
  pour Bottom (isolate 0.254): 0.76,-1.27 69.09,-1.27 arc90 71.12,0.76 71.12,52.58 arc90 69.09,54.61 0.76,54.61 arc90 -1.27,52.58 -1.27,0.76 arc90
  pour Top (isolate 0.254): 0.76,-1.27 69.09,-1.27 arc90 71.12,0.76 71.12,52.58 arc90 69.09,54.61 0.76,54.61 arc90 -1.27,52.58 -1.27,0.76 arc90
GPIO42  (via drill 0.25)
  Top 0.203: U26.1 3.26,36.62 R27.1
  Top 0.254: U26.1 4.56,36.62 v4.57,36.6
  Top 0.305: U$8.53 36.04,12.8 35.08,13.77 35.08,14.81 32.41,17.48 v32.41,20.34 | v27.28,20.37 27.28,24.64 v26.11,25.81
  Bottom 0.305: v32.41,20.34 27.3,20.34 v27.28,20.37 | v26.11,25.81 22.17,25.81 21.57,25.2 6.27,25.2 4.7,26.77 4.7,32.51 5.44,33.25 5.44,35.92 4.75,36.6 v4.57,36.6
HP_L  (via drill 0.25)
  Top 0.254: v10.77,28.14 10.77,28.16 C17.1 | v10.24,42.29 10.57,42.29 11.22,41.64 U5.31
  Top 0.406: C14.2 12.45,28.13 C13.1 C17.1 C18.2 9.08,28.13 8.76,27.81 8.76,26.04 10.17,24.63 J3.4
  Bottom 0.254: v10.24,42.29 10.24,40.18 9.83,39.78 9.83,37.64 10.39,37.08 10.39,35.76 9.53,34.9 9.53,32.05 10.77,30.81 v10.77,28.14
HP_R  (via drill 0.25)
  Top 0.254: C18.1 9.69,27.24 9.65,27.2 | v11.58,27.15 11.58,27.18 | U5.29 12.22,41.88 11.56,42.55 v11.25,42.55
  Top 0.406: C15.2 C19.2 9.91,27.11 C18.1 | J3.3 9.87,18.76 10.29,19.18 11.56,19.18 13.34,20.95 13.34,26.35 C14.1 12.64,26.86 12.57,26.8 12.26,27.11 C15.2 | C15.2 11.62,27.11 v11.58,27.15
  Bottom 0.254: v11.58,27.15 11.58,30.89 10.23,32.24 arc-45 10.08,32.59 10.08,34.49 11.07,35.48 11.07,37.11 10.31,37.87 10.31,39.52 10.82,40.03 10.82,42.11 v11.25,42.55
HRXD
  Top 0.406: R31.1 47.37,46.1 | 47.37,46.1 48.39,46.1 49.15,45.34 52.07,45.34 J7.2 | Q7.3 50.42,40.39 48.26,42.55 48.26,45.21 47.37,46.1
HTXD  (via drill 0.41)
  Top 0.406: Q8.3 55.75,41.66 J7.5
  Bottom 0.406: R32.1 47.12,44.58 49.02,42.67 52.83,42.67 53.34,43.18 J7.5
  other vias: 46.61,44.58
MIC_BIAS
  Top 0.203: U5.1 9.07,40.69 | 9.07,40.69 8.89,40.87 8.89,43.36 C24.2 | R8.2 7.34,39.45 8.58,40.69 9.07,40.69
MIC_N
  Top 0.254: C25.2 C49.2 | C48.2 C49.2 | C49.2 13.08,30.61 14.35,31.88 R11.1
MIC_P  (via drill 0.2, 0.25, 0.3)
  Top 0.203: C26.2 9.2,31.88 v8.71,32.36 | v7.29,36.45 7.29,38.33 v8.33,39.37 | v5.51,39.37 R8.1
  Top 0.254: C12.1 7.62,27.05 8.13,27.56 8.13,29.59 9.14,30.61 9.14,31.37 C26.2
  Top 0.406: R12.1 C12.1
  Bottom 0.152: 7.75,36.3 7.77,36.27
  Bottom 0.203: v8.71,32.36 8.15,32.92 8.15,35.89 7.77,36.27 | v8.33,39.37 v5.51,39.37 | v7.29,36.45 7.59,36.45 7.75,36.3
MRXD
  Top 0.406: J7.1 55.88,47.24 57.91,49.28 59.44,49.28 U3.2
MTXD
  Top 0.406: J7.6 56.77,44.07 57.28,44.58 57.28,47.37 58.42,48.51 62.61,48.51 63.5,49.4 U3.1
N$1  (via drill 0.41)
  Bottom 0.406: R19.2 18.77,49.91 19.33,49.35 19.33,43.51 18.2,42.38 U4.7
  other vias: 18.41,49.91
N$2
  Top 0.406: R6.2 R4.1
  Top 0.61: R4.1 53.72,11.05 U1.5
N$3
  Top 0.406: 6.35,44.2 Q3.3 5.79,45.01 R20.2
N$4
  Top 0.254: U5.27 13.22,42.07 12.97,42.33 12.43,42.33 11.96,42.8 11.96,43.18 C7.2
N$5  (via drill 0.41)
  Top 0.406: v17.65,46.86 R18.1
  Bottom 0.406: U4.3 16.93,46.14 v17.65,46.86
N$6  (via drill 0.41)
  Top 0.305: R17.1 17.2,48.39 16.56,47.75 16.56,45.26 18.52,43.31 18.52,41.17 v18.54,41.15
  Bottom 0.406: 16.6,41.11 U4.2 16.97,41.15 v18.54,41.15
N$7
  Top 0.406: D3.- 2.74,44.98 3.12,45.36 3.12,45.7 3.96,46.53 R20.1
N$8
  Top 0.406: Q3.1 R15.1 R13.2
N$9  (via drill 0.41)
  Top 0.305: R32.2 45.09,40.13 42.34,37.39 42.34,24.84 v46.23,20.95 | v51.18,21.34 D1.2
  Top 0.406: R31.2 R32.2 | D1.2 53.01,22.3 R7.1 C9.2 R9.2
  Bottom 0.305: v46.23,20.95 50.8,20.95 v51.18,21.34
N$11  (via drill 0.41)
  Top 0.406: 16.13,4.06 16.2,4 Q5.1 16.32,4.06 v16.38,4.06
  Bottom 0.406: v16.38,4.06 7.62,4.06 4.83,6.86 4.83,13.34 3.94,14.22 R22.1
  other vias: 3.17,14.22
N$12
  Bottom 0.61: P2.1 60.39,31.88 ANT1.2 ANT1.3 ANT1.4 ANT1.1
N$13  (via drill 0.25, 0.3)
  Top 0.254: U5.11 11.72,35.24 11.35,34.87 10.06,34.87 9.5,35.43 v9.5,36.04 | 6.58,37.95 U26.3 6.39,38.22 v6.45,38.15
  Bottom 0.254: v9.5,36.04 9.5,37.39 9.14,37.74 8.53,37.74 8.13,38.15 v6.45,38.15
N$14
  Top 0.406: R3.1 35.18,45.85 JP.2
N$15
  Top 0.406: R10.2 33.27,9.02 34.29,10.03 42.04,10.03 | C8.2 C6.2 41.27,6.6 42.04,7.37 42.04,10.03 | U$8.59 42.04,10.03
N$16
  Top 0.406: R21.2 6.1,48.51 Q4.3
N$17
  Top 0.406: D2.- R21.1
N$18
  Top 0.406: Q4.1 8.89,50.16 R16.1 R14.2
N$19
  Top 0.406: MAIN_ANTENNA.D 35.94,5.84 35.56,5.46 33.91,5.46 33.27,6.1 R10.1
N$20
  Top 0.406: R23.1 18.92,3.56 Q5.3
  Top 0.61: D6.+ 13.16,6.4 13.97,5.59 18.67,5.59 20.07,4.19 R23.1
N$21  (via drill 0.2)
  Top 0.203: v8.13,30.61 8,30.73 8,36.45 7.75,36.7 7.75,38.1 8.38,38.73 8.64,38.73 9.09,39.19 U5.4
  Top 0.254: C25.1 v9.91,30.35
  Bottom 0.203: v9.91,30.35 8.38,30.35 v8.13,30.61
N$22  (via drill 0.2)
  Top 0.203: C26.1 9.14,33.4 8.38,34.16 8.38,36.6 8.18,36.8 8.18,37.64 8.89,38.35 v9.27,38.35 | U5.3 9.21,39.69 v9.02,39.88
  Bottom 0.203: v9.27,38.35 9.27,39.62 v9.02,39.88
N$25
  Top 0.406: U21.4 1.37,42.84 2.08,43.56 C41.2
N$26
  Top 0.254: R25.1 4.41,42.67 U21.3
  Top 0.406: U21.3 3.97,42.19
N$28
  Top 0.254: U12.3 2.1,31.82 2.41,32.13 2.41,33.53 2.03,33.91 | U12.1 1.84,33.72 2.03,33.91 | R26.1 2.92,34.8 2.03,33.91
N$30
  Top 0.406: C16.2 R12.2 | 1.14,26.92 C16.2 | C16.2 1.65,26.67 1.65,18.87 3.53,17 J3.1
N$36
  Top 0.406: R3.2 R2.1 38.92,47.56 Q1.1
N$39
  Top 0.406: R22.2 R24.1 7.24,12.7 | 7.24,12.7 8.89,12.7 9.78,11.81 C22.1 | D4.2 7.25,12.72 7.24,12.7
N$53
  Top 0.406: PWR.- R1.1
N$54
  Top 0.406: U$8.79 51.18,35.18 C32.2
N$55
  Top 0.406: C32.1 53.59,35.56 55.88,35.56 GNSS_ANTENNA.D
NETLIGHT  (via drill 0.25, 0.41)
  Top 0.254: R13.1 10.41,44.91 v10.44,44.93
  Top 0.406: U$8.51 34.04,14.73 29.72,19.05 29.72,35.56 27.69,37.59 v26.42,37.59
  Bottom 0.254: v26.42,37.59 25.53,37.59 22.61,40.51 22.61,45.47 21.08,46.99 21.08,50.93 20.19,51.82 18.41,51.82 16.76,50.16 16.76,47.62 16.38,47.24 10.92,47.24 10.44,46.76 v10.44,44.93
PCM_CLK  (via drill 0.25)
  Top 0.254: v47.37,35.64 47.37,32.64 47.83,32.18 U$8.76 | v16.61,34.85 12.68,34.85 12.22,35.3 U5.12
  Bottom 0.254: v16.61,34.85 34.49,34.85 35.2,34.14 46.35,34.14 47.37,35.15 v47.37,35.64
PCM_DIN  (via drill 0.25)
  Top 0.254: U$8.74 46.81,30.18 45.74,31.24 v45.74,36.42 | U5.16 15.56,36.64 16.89,37.97 20.6,37.97 v21.51,38.89
  Bottom 0.254: v45.74,36.42 45.7,36.47 23.34,36.47 22.99,36.83 22.99,38.1 22.2,38.89 v21.51,38.89
PCM_DOUT  (via drill 0.25)
  Top 0.254: U$8.73 46.74,29.18 44.91,31.01 v44.91,35.64 | U5.14 13.22,36.08 13.44,35.87 15.54,35.87 17.14,37.47 21.13,37.47 v21.46,37.8
  Bottom 0.254: v44.91,35.64 35.48,35.64 35.18,35.94 22.86,35.94 22.23,36.58 22.23,37.47 21.89,37.8 v21.46,37.8
PCM_SYNC  (via drill 0.25)
  Top 0.254: U$8.75 47.45,31.18 46.79,31.85 46.79,35.03 v46.48,35.33 | v21.41,36.63 21.08,36.96 17.4,36.96 15.75,35.31 13.08,35.31 12.72,35.67 U5.13
  Bottom 0.254: 46.46,35.33 v46.48,35.33 46.3,35.15 46.3,35.13 46,34.82 35.41,34.82 34.8,35.43 21.97,35.43 21.46,35.94 21.46,36.58 v21.41,36.63
PWRKEY  (via drill 0.41)
  Top 0.406: Q1.3 42.29,45.21 40.94,43.86 U$8.3 40.94,20.02 45.21,15.75 v45.21,12.95 | K1.P$2 8.89,6.73 v12.95,10.79
  Bottom 0.406: v12.95,10.79 13.34,11.18 43.56,11.18 45.21,12.83 v45.21,12.95
RI  (via drill 0.41)
  Top 0.305: U$8.69 47.71,25.18 43.03,29.87 43.03,36.55 v46.35,39.88
  Bottom 0.305: v46.35,39.88 56.77,39.88 57.78,40.89 57.78,42.93 59.18,44.32 J1.2
RTS  (via drill 0.41)
  Top 0.305: U$8.66 46.9,22.18 v46.61,22.48
  Bottom 0.305: v46.61,22.48 46.61,31.37 49.53,34.29 59.82,34.29 60.83,35.31 J1.5
RXD  (via drill 0.3, 0.41)
  Top 0.305: U$8.68 47.44,24.18 v44.83,26.8 | v53.09,36.2 R30.2 | J1.7 63.37,38.99 62.36,37.97 58.42,37.97 v57.91,37.47
  Top 0.406: Q7.2 53.27,36.89 R30.2
  Bottom 0.305: v44.83,26.8 44.83,31.75 48.9,35.81 52.7,35.81 v53.09,36.2 53.47,35.81 57.28,35.81 57.91,36.45 v57.91,37.47
SCL  (via drill 0.25, 0.3)
  Top 0.254: U5.17 15.34,37.19 16.61,38.46 19.53,38.46 20.83,39.75 24.64,39.75 25.65,38.73 28.45,38.73 v29.97,40.26
  Top 0.305: v37.59,39.24 37.59,16.26 38.1,15.75 38.1,11.44 U$8.55
  Bottom 0.254: v29.97,40.26 29.97,43.31 28.57,44.7 28.57,46.74 29.21,47.37 31.37,47.37 32,46.74 R29.1
  Bottom 0.305: R29.1 32,43.81 32.89,42.93 36.2,42.93 37.59,41.53 v37.59,39.24
  other vias: 32,45.97
SDA  (via drill 0.25, 0.3)
  Top 0.254: U5.18 15.11,37.69 16.36,38.94 19,38.94 20.32,40.26 25.02,40.26 25.78,39.5 27.81,39.5 v28.7,40.39 | v28.7,43.43 28.7,45.21 29.46,45.97 R28.1
  Top 0.305: v39.62,37.34 39.62,13.59 38.99,12.95 38.99,11.44 U$8.56
  Bottom 0.254: v28.7,40.39 v28.7,43.43
  Bottom 0.305: R28.1 30.1,44.58 32.38,42.29 35.43,42.29 36.7,41.02 36.7,37.85 37.21,37.34 v39.62,37.34
  other vias: 30.1,45.97
SIM_CLK
  Top 0.305: R18.2 21.46,46.86 24.94,43.38 U$8.19
SIM_DATA
  Top 0.305: R19.1 20.7,49.91 24.13,46.48 25.53,46.48 26.94,45.07 U$8.17
SIM_RST
  Top 0.305: R17.2 21.34,48.39 25.94,43.78 U$8.18
SIM_VDD  (via drill 0.41)
  Top 0.305: C20.1 21.84,45.34 23.94,43.24 U$8.20
  Top 0.406: v20.19,42.95 20.19,45.09 C20.1
  Bottom 0.406: U4.1 17.36,38.57 17.4,38.61 19.43,38.61 20.19,39.37 v20.19,42.95
SRXD
  Top 0.406: J7.3 50.55,46.61 49.4,47.75 44.7,47.75 U3.9
STATUS  (via drill 0.3, 0.41)
  Top 0.305: R14.1 11.38,48.51 12.19,49.33 12.19,50.11 12.78,50.7 17.42,50.7 17.78,51.05 v19.1,51.05 | v28.83,32.26 28.83,34.29 27.94,35.18 25.91,35.18 24.26,36.83 v24.26,37.47
  Top 0.406: U$8.49 32.04,14.95 28.83,18.16 v28.83,32.26
  Bottom 0.254: v19.1,51.05 19.56,51.05 20.32,50.29 20.32,46.48 21.97,44.83 21.97,40.39 24.26,38.1 v24.26,37.47
STXD
  Bottom 0.406: J7.4 49.28,44.07 48.51,44.83 48.51,46.61 45.72,49.4 U3.8
TXD
  Top 0.305: Q8.2 56.7,38.8 58.42,40.51 62.36,40.51 63.37,41.53 J1.8
  Top 0.406: U$8.71 51.68,27.18 52.32,26.54 55.75,26.54 56.52,27.3 56.52,29.46 56.77,29.72 62.36,29.72 63.12,30.48 63.12,33.15 61.85,34.42 59.69,34.42 57.28,36.83 R33.1 56.52,38.17 Q8.2
USB_DN  (via drill 0.41)
  Top 0.381: J6.2 6.84,8.14
  Top 0.406: 6.84,8.14 v6.86,8.13 | v31.88,26.16 31.88,41.92 U$8.12
  Bottom 0.406: v6.86,8.13 7.62,8.89 7.62,21.34 9.65,23.37 27.3,23.37 29.46,25.53 31.24,25.53 v31.88,26.16
USB_DP  (via drill 0.41)
  Top 0.381: J6.3 6.1,7.49 v6.73,6.86
  Top 0.406: v30.73,24.38 30.73,28.57 30.99,28.83 30.99,41.94 U$8.13
  Bottom 0.406: v6.73,6.86 7.24,6.86 8.64,8.26 8.64,20.95 10.16,22.48 29.46,22.48 30.73,23.75 v30.73,24.38
USB_VBUS  (via drill 0.41)
  Top 0.381: J6.1 5.75,8.79 v6.1,9.14
  Top 0.406: v33.02,29.08 33.02,41.91 U$8.11
  Bottom 0.406: v33.02,29.08 30.48,26.54 28.96,26.54 26.67,24.26 9.4,24.26 6.1,20.95 v6.1,9.14
VBAT  (via drill 0.25, 0.3, 0.41)
  Top 0.203: C40.2 7.09,41.15 7.14,41.2 | v13.92,42.09 13.92,41.91 13.89,41.88 13.87,41.88 13.86,41.87 | v8.28,42.29 7.37,42.29 R25.2
  Top 0.254: C44.2 1.14,30.35 0.43,31.06 0.43,32.79 | 0.43,32.79 0.43,34.47 R26.2 1.22,35.43 0.58,36.07 0.58,39.32 0.71,39.45 3.73,39.45 3.97,39.68 U21.1 6.8,40.33 6.99,40.51 C40.2 | U12.2 0.46,32.77 0.43,32.79 | U5.26 13.72,41.74 13.86,41.87 13.89,41.91 14.55,41.91 16.03,40.44 C37.2 | C35.2 15.52,45.06 17.3,43.28 C36.2 17.3,41.35 C37.2 | U5.21 15.57,39.19 16.03,39.65 C37.2
  Top 0.305: C35.2 15.52,47.73 C34.2
  Top 0.406: C30.+ 14.61,16.7 | 14.61,16.7 13.65,16.7 13.34,16.38 13.34,14.99 C31.2 | R25.2 C40.2 | v4.83,21.59 11.56,21.59 v11.81,21.34 | v14.22,18.92 14.22,17.08 14.61,16.7
  Top 0.61: C5.2 56.77,8.51 | 56.77,8.51 56.77,12.32 55.5,13.59 U1.4 50.29,13.59 | R5.2 C5.2 | VBAT.1 63.75,6.1 61.34,8.51 56.77,8.51 | C5.2 R4.2 | U$8.38 U$8.39 16.02,18.18 15.11,17.27 C30.+ 15.68,16.7 18.92,13.46 v18.92,10.03 | U$8.63 U$8.62 49.89,18.18 50.29,17.78 50.29,13.59 | 50.29,13.59 50.29,10.54 49.4,9.65 C28.+ 48.2,9.21 47.5,8.51 47.5,7.11 47.12,6.73 C11.2 C10.2 44.2,5.21 43.43,4.45 31.24,4.45 29.78,2.98 29.78,3.11 C4.+ v28.96,3.94
  Bottom 0.203: v13.92,42.09 13.23,42.09 12.12,43.2 9.2,43.2 v8.28,42.29
  Bottom 0.406: C44.2 1.27,23.11 2.54,21.84 4.57,21.84 v4.83,21.59 | v11.81,21.34 v14.22,18.92
  Bottom 0.61: v28.96,3.94 22.23,3.94 18.92,7.24 v18.92,10.03
  other vias: 1.27,30.35
VDD_EXT  (via drill 0.25, 0.41)
  Top 0.254: v38.48,38.12 38.48,19.74 v38.43,19.68
  Top 0.305: v51.44,38.35 51.44,38.99 51.82,39.37 54.48,39.37 54.74,39.12 54.74,38.42 Q8.1 v54.86,38.35
  Top 0.406: R30.1 51.37,36.89 Q7.1 v51.44,38.35 | Q8.1 54.8,37.02 R33.2 | U$8.44 27.04,12.31 v27.69,12.95
  Bottom 0.254: v51.44,38.35 38.71,38.35 v38.48,38.12
  Bottom 0.305: J1.9 63.37,43.94 62.48,43.05 59.18,43.05 58.55,42.42 58.55,40.13 56.77,38.35 v54.86,38.35 | v27.69,12.95 32.51,12.95 38.43,18.87 v38.43,19.68
  Bottom 0.406: J1.10 J1.9
VIN  (via drill 0.3, 0.41)
  Top 0.406: D3.+ D2.+ 1.4,48.51 1.02,48.9 1.02,51.31 1.27,51.56 PWR.+
  Top 0.61: C3.+ 60.13,23.69 58.67,25.15 56.52,25.15 56.13,24.77 C1.2 C2.2 54.61,22.35 R7.2 54.55,20.13 52.96,18.54 U1.1 U1.2 v54.99,16.89 | v20.19,9.27 20.19,7.92 D5.- | D6.- 17.58,8.46 15.75,10.29 v15.75,12.19 | v15.75,19.94 v15.75,26.52 | PWR.+ 2.03,52.07 2.67,52.7 20.19,52.7 21.72,51.18 21.72,49.91 23.75,47.88 26.64,47.88 v27.36,47.17 | v34.92,31.11 34.92,39.29 v34.85,39.37
  Top 0.813: D5.- D6.-
  Bottom 0.61: v54.99,16.89 54.99,15.37 49.53,9.91 20.83,9.91 v20.19,9.27 | v15.75,12.19 v15.75,19.94 | v15.75,26.52 15.75,26.67 16.38,27.3 24.26,27.3 27.43,30.48 34.29,30.48 v34.92,31.11 | v34.85,39.37 28.45,39.37 27.43,40.39 27.43,47.09 v27.36,47.17
VRTC  (via drill 0.41)
  Top 0.406: C29.2 26.8,8.76 25.04,10.52 U$8.42 25.04,14.33 v25.02,14.35
  Bottom 0.406: v25.02,14.35 25.02,14.41 J14.+

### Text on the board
tPlace: GPRS_RX | Status | SWserial | GND | VDD_EXT | Xduino | RI | NetLight | GPRS_TX | DCD | TXD | CTS | RXD | RTS | DTR | GND | 4.2V
bPlace: SIM Card Holder | SIM5360E GSM GPS 3G shield | v1.0 04/08/2017 | www.elecrow.com | 3V CR1220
